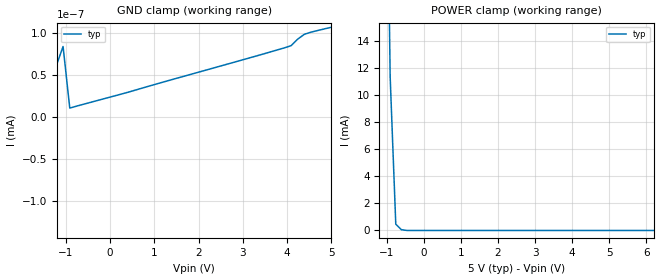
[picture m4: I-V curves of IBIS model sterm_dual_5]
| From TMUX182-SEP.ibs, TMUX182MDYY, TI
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| sterm_dual_5
[Model]   sterm_dual_5
Model_type   Terminator
|   typ   min   max
C_comp   4.014581e-12   NA   NA
[Voltage Range]   5   NA   NA
[Temperature Range]   27   NA   NA
[Power Clamp Reference]   5   NA   NA
[GND Clamp Reference]   0   NA   NA
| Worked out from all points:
|   GND clamp passes 1 mA (typ) near -5.76 V on its own axis
|   POWER clamp passes 1 mA (typ) near -0.76 V on its own axis
[GND Clamp]
|   Voltage   I(typ)   I(min)   I(max)
-10V      -2.321A    NA         NA
-5.455V   -30.47nA   NA         NA
-5.303V   -84.49pA   NA         NA
-5.152V   -60.21pA   NA         NA
-3.939V   -34.13pA   NA         NA
-2.424V   -11.7pA    NA         NA
-2.273V   -94.68pA   NA         NA
-1.061V   83.87pA    NA         NA
-909.1mV  10.66pA    NA         NA
3.939V    82.28pA    NA         NA
4.394V    98.48pA    NA         NA
5V        106.8pA    NA         NA
[POWER Clamp]
|   Voltage   I(typ)   I(min)   I(max)
-5V       1.914A     NA         NA
-1.061V   43.19mA    NA         NA
-909.1mV  11.39mA    NA         NA
-757.6mV  467.9uA    NA         NA
-606.1mV  57.26uA    NA         NA
-303mV    751pA      NA         NA
10V       -58.08pA   NA         NA
